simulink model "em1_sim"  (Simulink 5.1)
settings: Solver=ode45  StartTime=Ts  StopTime=Te  RelTol=1e-3
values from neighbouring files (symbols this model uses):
  em1_co0 = O_0    [simulateEM1m.m]
  em1_coin = O_in    [simulateEM1m.m]
  em1_cs0 = S_0    [simulateEM1m.m]
  em1_csin = S_in    [simulateEM1m.m]
  em1_cx0 = X_0    [simulateEM1m.m]
  em1_Ki = Ki    [simulateEM1m.m]
  em1_kla = kla    [simulateEM1m.m]
  em1_Ks = Ks    [simulateEM1m.m]
  em1_Osat = O_sat    [simulateEM1m.m]
  em1_qin = q_in    [simulateEM1m.m]
  em1_sample = h / (60 * 60)    [simulateEM1m.m]
  em1_V0 = V_0    [simulateEM1m.m]

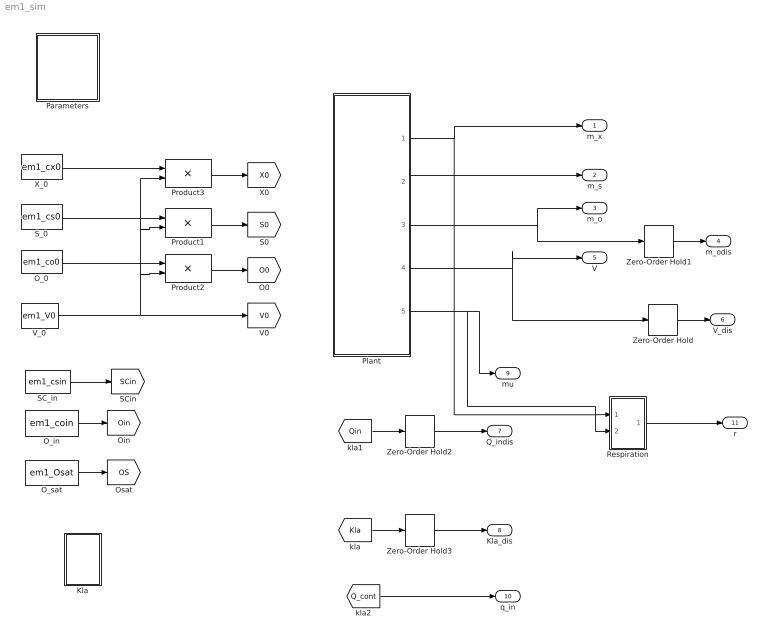
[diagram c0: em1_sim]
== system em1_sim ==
  Kla : Subsystem
  O_0 : Constant  Value=em1_co0
  O_in : Constant  Value=em1_coin
  O_sat : Constant  Value=em1_Osat
  Parameters : Subsystem
  Plant : Subsystem
  Product1 : Product
  Product2 : Product
  Product3 : Product
  Respiration : Subsystem
  SC_in : Constant  Value=em1_csin
  S_0 : Constant  Value=em1_cs0
  V_0 : Constant  Value=em1_V0
  X_0 : Constant  Value=em1_cx0
  Zero-Order Hold{,1..3} (4 alike) : ZeroOrderHold  SampleTime=em1_sample
  m_x : Outport
  m_s : Outport  Port=2
  m_o : Outport  Port=3
  m_odis : Outport  Port=4
  V : Outport  Port=5
  V_dis : Outport  Port=6
  Q_indis : Outport  Port=7
  Kla_dis : Outport  Port=8
  mu : Outport  Port=9
  q_in : Outport  Port=10
  r : Outport  Port=11
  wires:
  V_0/1 -> [V0], Product1/2, Product3/2, Product2/2
  O_sat/1 -> [OS]
  SC_in/1 -> [SCin]
  O_in/1 -> [Oin]
  Product1/1 -> [S0]
  S_0/1 -> Product1/1
  Product2/1 -> [O0]
  O_0/1 -> Product2/1
  X_0/1 -> Product3/1
  Product3/1 -> [X0]
  Plant/1(m_x) -> m_x/1, Respiration/1(mx)
  Plant/2(m_s) -> m_s/1
  Plant/3(m_o) -> m_o/1, Zero-Order Hold1/1
  Plant/4(V) -> V/1, Zero-Order Hold/1
  Zero-Order Hold1/1 -> m_odis/1
  Zero-Order Hold/1 -> V_dis/1
  Plant/5(mu) -> mu/1, Respiration/2(mu)
  [Kla] -> Zero-Order Hold3/1
  Zero-Order Hold3/1 -> Kla_dis/1
  [Qin] -> Zero-Order Hold2/1
  Zero-Order Hold2/1 -> Q_indis/1
  [Q_cont] -> q_in/1
  Respiration/1(r) -> r/1

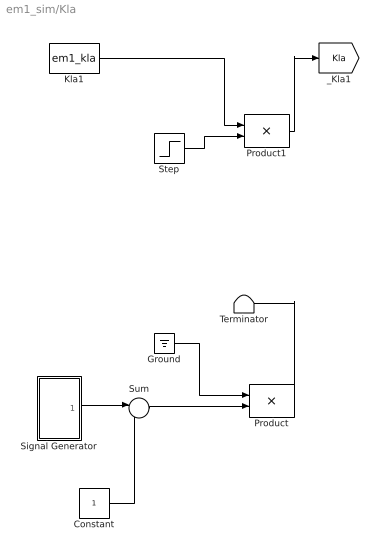
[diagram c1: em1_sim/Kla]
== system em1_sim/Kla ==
  Constant : Constant
  Ground : Ground
  Kla1 : Constant  Value=em1_kla
  Product : Product
  Product1 : Product
  Signal Generator : Subsystem
  Step : Step  Time=0.8  Before=1  SampleTime=em1_sample
  Sum : Sum  Inputs=|-+
  Terminator : Terminator
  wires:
  Signal Generator/1(rnd_rec) -> Sum/1
  Sum/1 -> Product/2
  Constant/1 -> Sum/2
  Product/1 -> Terminator/1
  Ground/1 -> Product/1
  Step/1 -> Product1/2
  Kla1/1 -> Product1/1
  Product1/1 -> [Kla]

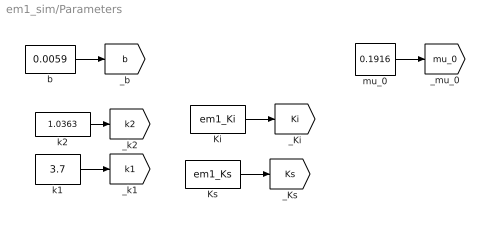
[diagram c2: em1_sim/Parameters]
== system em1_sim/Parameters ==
  Ki : Constant  Value=em1_Ki
  Ks : Constant  Value=em1_Ks
  b : Constant  Value=0.0059
  k1 : Constant  Value=3.7
  k2 : Constant  Value=1.0363
  mu_0 : Constant  Value=0.1916
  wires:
  b/1 -> [b]
  k2/1 -> [k2]
  k1/1 -> [k1]
  mu_0/1 -> [mu_0]
  Ks/1 -> [Ks]
  Ki/1 -> [Ki]

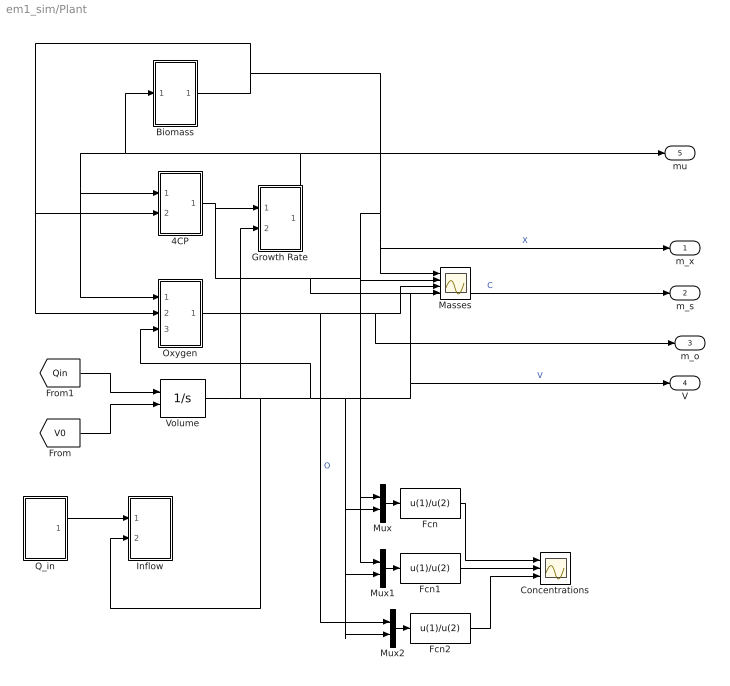
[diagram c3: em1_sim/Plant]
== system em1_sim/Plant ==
  4CP : Subsystem
  Biomass : Subsystem
  Concentrations : Scope  NumInputPorts=3
  Fcn : Fcn  Expr=u(1)/u(2)
  Fcn1 : Fcn  Expr=u(1)/u(2)
  Fcn2 : Fcn  Expr=u(1)/u(2)
  Growth Rate : Subsystem
  Inflow : Subsystem
  Masses : Scope  NumInputPorts=4
  Mux : Mux  Inputs=2
  Mux1 : Mux  Inputs=2
  Mux2 : Mux  Inputs=2
  Oxygen : Subsystem
  Q_in : Subsystem
  Volume : Integrator  InitialConditionSource=external
  m_x : Outport
  m_s : Outport  Port=2
  m_o : Outport  Port=3
  V : Outport  Port=4
  mu : Outport  Port=5
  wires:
  [V0] -> Volume/2
  Volume/1 -> Oxygen/3(V), Mux/2, Mux1/2, Mux2/2, V/1, Masses/4, Inflow/2(V), Growth Rate/2(V)  "V"
  [Qin] -> Volume/1
  Growth Rate/1(mu) -> Oxygen/1(mu), 4CP/1(mu), Biomass/1(mu), mu/1
  Biomass/1(X) -> Oxygen/2(X), 4CP/2(X), Mux/1, Masses/1, m_x/1  "X"
  Oxygen/1(O) -> Mux2/1, Masses/3, m_o/1  "O"
  Q_in/1(q_in) -> Inflow/1(Q_in)
  4CP/1(4CP) -> Growth Rate/1(CP4), Mux1/1, Masses/2, m_s/1  "C"
  Fcn/1 -> Concentrations/1
  Fcn1/1 -> Concentrations/2
  Fcn2/1 -> Concentrations/3
  Mux/1 -> Fcn/1
  Mux1/1 -> Fcn1/1
  Mux2/1 -> Fcn2/1

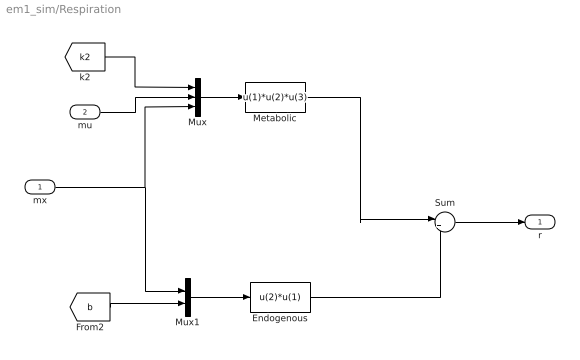
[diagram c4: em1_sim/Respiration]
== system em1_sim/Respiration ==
  mx : Inport
  mu : Inport  Port=2
  Endogenous : Fcn  Expr=u(2)*u(1)
  Metabolic : Fcn  Expr=u(1)*u(2)*u(3)
  Mux : Mux  Inputs=3
  Mux1 : Mux  Inputs=2
  Sum : Sum  Inputs=|++
  r : Outport
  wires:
  [k2] -> Mux/1
  Mux/1 -> Metabolic/1
  mu/1 -> Mux/2
  mx/1 -> Mux/3, Mux1/1
  [b] -> Mux1/2
  Mux1/1 -> Endogenous/1
  Metabolic/1 -> Sum/1
  Endogenous/1 -> Sum/2
  Sum/1 -> r/1

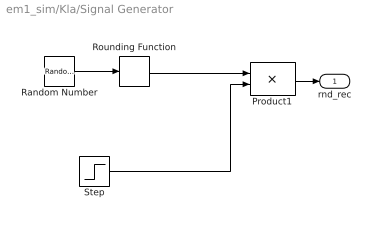
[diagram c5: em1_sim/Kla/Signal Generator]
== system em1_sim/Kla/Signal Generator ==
  Product1 : Product
  Random Number : RandomNumber  Mean=1  SampleTime=0
  Rounding Function : Rounding
  Step : Step  Time=0  SampleTime=0
  rnd_rec : Outport
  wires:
  Random Number/1 -> Rounding Function/1
  Step/1 -> Product1/2
  Rounding Function/1 -> Product1/1
  Product1/1 -> rnd_rec/1

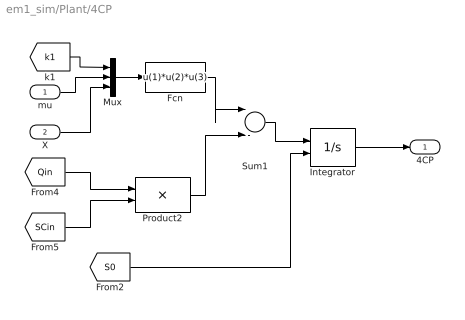
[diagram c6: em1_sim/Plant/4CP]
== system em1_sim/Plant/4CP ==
  mu : Inport
  X : Inport  Port=2
  Fcn : Fcn  Expr=u(1)*u(2)*u(3)
  Integrator : Integrator  InitialConditionSource=external
  Mux : Mux  Inputs=3
  Product2 : Product
  Sum1 : Sum  Inputs=|-+
  4CP : Outport
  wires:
  X/1 -> Mux/3
  mu/1 -> Mux/2
  [k1] -> Mux/1
  Mux/1 -> Fcn/1
  Integrator/1 -> 4CP/1
  [S0] -> Integrator/2
  [Qin] -> Product2/1
  [SCin] -> Product2/2
  Fcn/1 -> Sum1/1
  Product2/1 -> Sum1/2
  Sum1/1 -> Integrator/1

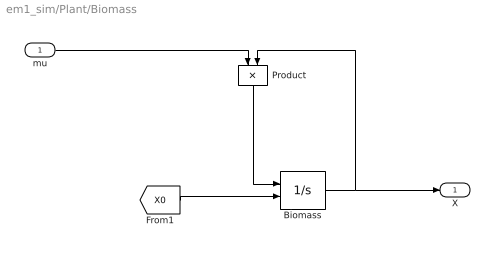
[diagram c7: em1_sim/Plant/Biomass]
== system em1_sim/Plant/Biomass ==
  mu : Inport
  Biomass : Integrator  InitialConditionSource=external
  Product : Product  Orientation=down
  X : Outport
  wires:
  Product/1 -> Biomass/1
  mu/1 -> Product/1
  Biomass/1 -> X/1, Product/2
  [X0] -> Biomass/2

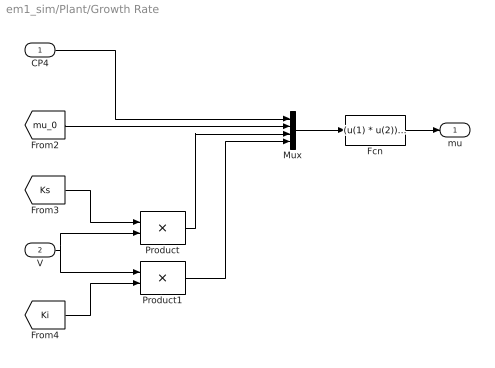
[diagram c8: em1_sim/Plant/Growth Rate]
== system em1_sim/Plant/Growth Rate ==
  CP4 : Inport
  V : Inport  Port=2
  Fcn : Fcn  Expr=(u(1) * u(2))/(u(3) + u(1) + (u(1)^2/u(4)))
  Mux : Mux
  Product : Product
  Product1 : Product
  mu : Outport
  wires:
  Mux/1 -> Fcn/1
  CP4/1 -> Mux/1
  Fcn/1 -> mu/1
  [mu_0] -> Mux/2
  V/1 -> Product/2, Product1/1
  [Ks] -> Product/1
  Product/1 -> Mux/3
  [Ki] -> Product1/2
  Product1/1 -> Mux/4

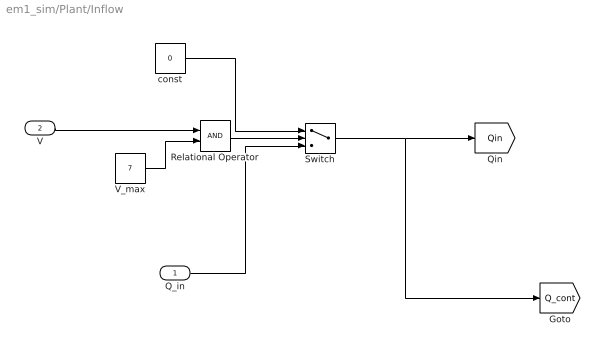
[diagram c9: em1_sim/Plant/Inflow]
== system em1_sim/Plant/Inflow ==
  Q_in : Inport
  V : Inport  Port=2
  Relational Operator : RelationalOperator  ShowAdditionalParam=on  SampleTime=em1_sample
  Switch : Switch  Criteria=u2 ~= 0  ShowAdditionalParam=on  SampleTime=em1_sample
  V_max : Constant  Value=7
  const : Constant  Value=0
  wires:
  Switch/1 -> [Qin], [Q_cont]
  V_max/1 -> Relational Operator/2
  V/1 -> Relational Operator/1
  Relational Operator/1 -> Switch/2
  const/1 -> Switch/1
  Q_in/1 -> Switch/3

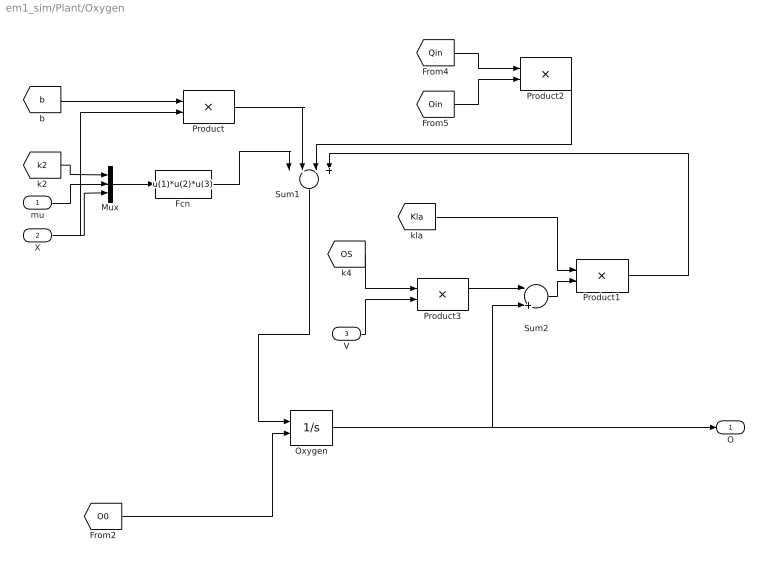
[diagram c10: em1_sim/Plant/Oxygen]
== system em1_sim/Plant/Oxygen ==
  mu : Inport
  X : Inport  Port=2
  V : Inport  Port=3
  Fcn : Fcn  Expr=u(1)*u(2)*u(3)
  Mux : Mux  Inputs=3
  Oxygen : Integrator  InitialConditionSource=external
  Product{,1..3} (4 alike) : Product
  Sum1 : Sum  Orientation=down  Inputs=|--++
  Sum2 : Sum  Inputs=|+-
  O : Outport
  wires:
  Sum1/1 -> Oxygen/1
  Sum2/1 -> Product1/2
  Product1/1 -> Sum1/4
  Product/1 -> Sum1/2
  [O0] -> Oxygen/2
  Oxygen/1 -> Sum2/2, O/1
  Fcn/1 -> Sum1/1
  X/1 -> Product/2, Mux/3
  mu/1 -> Mux/2
  [k2] -> Mux/1
  Mux/1 -> Fcn/1
  [b] -> Product/1
  [Qin] -> Product2/1
  [Oin] -> Product2/2
  Product2/1 -> Sum1/3
  [Kla] -> Product1/1
  Product3/1 -> Sum2/1
  [OS] -> Product3/1
  V/1 -> Product3/2

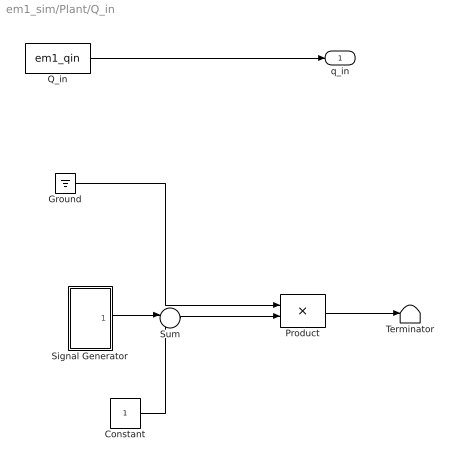
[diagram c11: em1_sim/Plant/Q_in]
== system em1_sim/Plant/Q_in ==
  Constant : Constant
  Ground : Ground
  Product : Product
  Q_in : Constant  Value=em1_qin
  Signal Generator : Subsystem
  Sum : Sum  Inputs=|-+
  Terminator : Terminator
  q_in : Outport
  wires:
  Constant/1 -> Sum/2
  Sum/1 -> Product/2
  Signal Generator/1(rnd_rec) -> Sum/1
  Ground/1 -> Product/1
  Product/1 -> Terminator/1
  Q_in/1 -> q_in/1

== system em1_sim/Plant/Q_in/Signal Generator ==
  Product1 : Product
  Random Number : RandomNumber  Mean=1  SampleTime=0
  Rounding Function : Rounding
  Step : Step  Time=0  SampleTime=0
  rnd_rec : Outport
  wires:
  Product1/1 -> rnd_rec/1
  Rounding Function/1 -> Product1/1
  Step/1 -> Product1/2
  Random Number/1 -> Rounding Function/1
